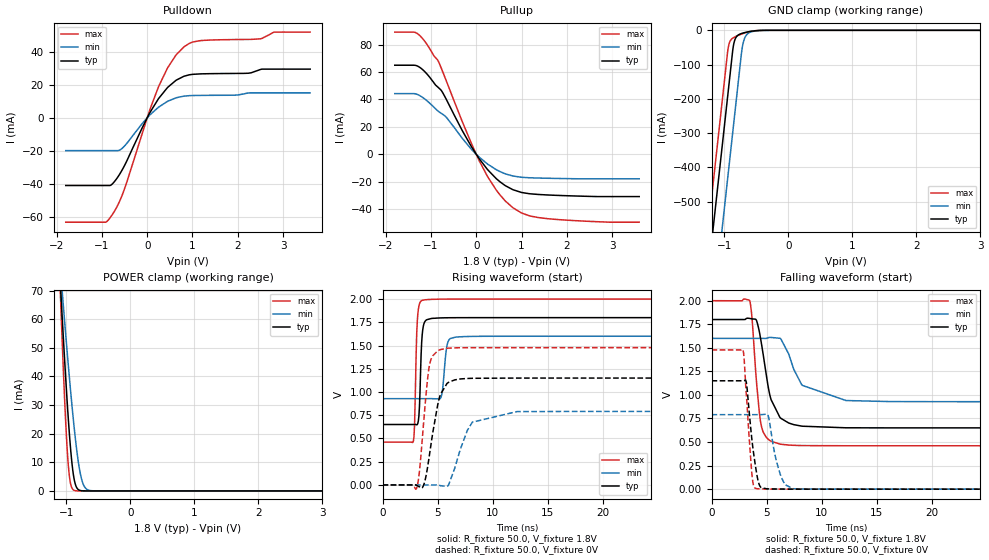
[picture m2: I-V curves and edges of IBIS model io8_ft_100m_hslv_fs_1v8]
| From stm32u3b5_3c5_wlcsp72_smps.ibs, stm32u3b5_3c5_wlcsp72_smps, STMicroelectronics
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[Model]   io8_ft_100m_hslv_fs_1v8
Model_type I/O
Polarity   Non-Inverting
Enable   Active-Low
| CAP_THRESHOLD on pad IOFT is "UDTCAPC" :
| Rising=30.0% of vddiom   Falling=70.0% of vddiom
| C_comp min and max val. don't necessarily correlate with the min and max pvt
| but are the smallest and greatest pad capacitance found.
| var   typ   min   max
C_comp   3.41787pF  3.41663pF  3.48192pF
|C_comp_pullup   1.92554pF  1.84326pF  2.10232pF
|C_comp_pulldown   1.49232pF  1.57337pF  1.37960pF
Vinl = 800.0mV
Vinh = 1.0V
Vmeas = 900.0mV   | Reference voltage for timing measurements
Cref  = 50.0pF   | Timing specification test load capacitance value
Rref  = 1.0MOhm   | Timing specification test load resistance value
Vref  = 990.0mV   | Timing specification test load voltage
[Model Spec]
| TIME_THRESHOLD on pin ZIV11 is "CMOS" :
| Rising=50.0% of vdd   Falling=50.0% of vdd
Vinl 694.50000mV 619.50000mV 778.50000mV
Vinh 1.08350V 957.50000mV 1.18750V
| variable   typ   min   max
[Temperature Range] 25.0 130.0 -40.0
| variable   typ   min   max
[Voltage Range] 1.8V 1.6V 2.0V
| variable   typ   min   max
[POWER Clamp Reference] 1.8V 1.6V 2.0V
| variable   typ   min   max
[GND Clamp Reference] 0V 0V 0V
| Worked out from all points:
|   slope of the pulldown table from 0 to 0.27 V, typ, clamps not added: 21.9 ohm
|   slope of the pullup table from 0 to 0.27 V, typ, clamps not added: 22.8 ohm
|   GND clamp passes 1 mA (typ) near -0.50 V on its own axis
|   POWER clamp passes 1 mA (typ) near -0.83 V on its own axis
|   rising waveform, R_fixture 50.0, V_fixture 1.8V: 20-80 % time 210ps typ, 321ps min, 196ps max; typ from 0.65 V to 1.8 V
|   falling waveform, R_fixture 50.0, V_fixture 1.8V: 20-80 % time 1.21ns typ, 2.33ns min, 635ps max; typ from 1.8 V to 0.65 V
|   rising waveform, R_fixture 50.0, V_fixture 0V: 20-80 % time 982ps typ, 1.45ns min, 660ps max; typ from 0 V to 1.15 V
|   falling waveform, R_fixture 50.0, V_fixture 0V: 20-80 % time 669ps typ, 867ps min, 510ps max; typ from 1.15 V to 0 V
[POWER Clamp]
-1.8V     399.1mA    292.1mA    557.7mA
-1.09V    71.2mA     76.8mA     67.14mA
-1.08V    67.05mA    73.98mA    61.2mA
-1.06V    58.89mA    68.38mA    49.67mA
-1.02V    43.22mA    57.4mA     28.67mA
-980mV    28.81mA    46.77mA    12.28mA
-940mV    16.45mA    36.61mA    3.257mA
-880mV    4.35mA     22.67mA    225.4uA
-820mV    610.4uA    11.29mA    13uA
-770mV    97.5uA     4.87mA     1.193uA
-640mV    753.9nA    196uA      2.492nA
3.6V      0A         0A         0A
[GND Clamp]
-1.8V     -1.64A     -1.88A     -1.509A
-1.24V    -688.2mA   -927.9mA   -557mA
-1.05V    -365.2mA   -604.9mA   -234mA
-950mV    -195.2mA   -434.9mA   -64mA
-930mV    -161.2mA   -400.9mA   -41.59mA
-870mV    -59.19mA   -298.9mA   -22.94mA
-850mV    -36.73mA   -264.9mA   -20.65mA
-770mV    -12.21mA   -128.9mA   -13.73mA
-730mV    -9.139mA   -62.1mA    -10.81mA
-690mV    -6.97mA    -26.33mA   -8.198mA
-530mV    -1.564mA   -2.413mA   -1.407mA
3.6V      1.228nA    159.5nA    526.9pA
| variable   typ   min   max
[Pullup Reference] 1.8V 1.6V 2.0V
| variable   typ   min   max
[Pulldown Reference] 0V 0V 0V
[Pullup]
-1.8V     64.92mA    44.22mA    89.08mA
-1.3V     64.34mA    43.62mA    87.96mA
-1.13V    59.98mA    40.13mA    82.03mA
-850mV    49.04mA    31.68mA    68.55mA
-670mV    40.59mA    27.29mA    54.24mA
-310mV    17.35mA    11.71mA    23.94mA
70mV      -3.42mA    -2.198mA   -4.946mA
440mV     -17.67mA   -11.15mA   -25.97mA
810mV     -25.79mA   -15.81mA   -38.95mA
1.18V     -28.75mA   -17.1mA    -44.89mA
1.56V     -29.61mA   -17.45mA   -46.86mA
3.6V      -30.8mA    -17.88mA   -49.48mA
[Pulldown]
-1.8V     -41.16mA   -19.96mA   -63.43mA
-920mV    -41.16mA   -19.96mA   -63.43mA
-780mV    -40.43mA   -19.96mA   -59.18mA
-510mV    -29.46mA   -17.38mA   -43.8mA
0V        0A         -230fA     0A
250mV     11.64mA    6.428mA    18.87mA
460mV     18.67mA    10.12mA    30.76mA
810mV     25.21mA    13.14mA    43.03mA
1.18V     26.67mA    13.59mA    46.9mA
2.5V      29.31mA    15.12mA    47.95mA
2.81V     29.55mA    15.12mA    52.03mA
3.6V      29.55mA    15.12mA    52.05mA
[Ramp]
dV/dt_r 690.0298mV/981.32916ps 474.38109mV/1.40579ns 886.36843mV/658.85282ps
dV/dt_f 689.75447mV/1.12579ns 403.00076mV/1.68065ns 923.68055mV/633.67172ps
R_load = 50.0
| Removed startup time: 0s 0s 0s  .
| Removed end time: 36.25ns.
[Rising Waveform]
R_fixture   = 50.0
V_fixture   = 1.8V
V_fixture_min = 1.6V
V_fixture_max = 2.0V
0s        650.4mV    928.3mV    460.5mV
2.8ns     650.7mV    928.3mV    473mV
2.9ns     650.8mV    928.3mV    632mV
3.15ns    649.8mV    928.3mV    1.755V
3.35ns    842.4mV    928.3mV    1.948V
3.6ns     1.617V     928.3mV    1.986V
5.25ns    1.797V     930.7mV    1.999V
5.9ns     1.799V     1.525V     2V
6.65ns    1.8V       1.591V     2V
36.25ns   1.8V       1.6V       2V
| Removed startup time: 0s 0s 0s  .
| Removed end time: 199.25ns.
[Falling Waveform]
R_fixture   = 50.0
V_fixture   = 1.8V
V_fixture_min = 1.6V
V_fixture_max = 2.0V
0s        1.8V       1.6V       2V
3.45ns    1.812V     1.6V       2.003V
3.65ns    1.808V     1.6V       1.842V
4.05ns    1.797V     1.6V       1.178V
4.55ns    1.527V     1.6V       655.8mV
5.4ns     950.1mV    1.61V      508.8mV
7ns       702mV      1.435V     468mV
8.25ns    668mV      1.101V     462.5mV
16.25ns   650.5mV    929.4mV    460.5mV
199.3ns   650.4mV    928.3mV    460.5mV
| Removed startup time: 0s 0s 0s  .
| Removed end time: 199.2ns.
[Rising Waveform]
R_fixture   = 50.0
V_fixture   = 0V
V_fixture_min = 0V
V_fixture_max = 0V
0s        4.636nV    97.72nV    3.408nV
3.05ns    -1.213mV   -226.6nV   -44.13mV
3.3ns     -17.75mV   -1.125uV   96.7mV
3.7ns     -9.956mV   -9.028uV   631mV
4.3ns     357.9mV    -18.37uV   1.312V
5.15ns    933.4mV    -2.891mV   1.452V
6ns       1.105V     2.808mV    1.472V
8.15ns    1.148V     675.6mV    1.477V
12.2ns    1.15V      789.4mV    1.477V
199.2ns   1.15V      790.6mV    1.477V
| Removed startup time: 0s 0s 0s  .
| Removed end time: 36.25ns.
[Falling Waveform]
R_fixture   = 50.0
V_fixture   = 0V
V_fixture_min = 0V
V_fixture_max = 0V
0s        1.15V      790.6mV    1.477V
2.85ns    1.15V      790.6mV    1.481V
3.15ns    1.136V     790.6mV    1.007V
3.65ns    536.3mV    790.6mV    171.8mV
4.05ns    195.9mV    790.7mV    6.559mV
4.4ns     30.04mV    790.7mV    3.072mV
5.1ns     3.457mV    790.2mV    1.414mV
6.3ns     1.163mV    133.8mV    471.6uV
7.4ns     526uV      4.771mV    194.6uV
36.25ns   48.37nV    588.8nV    5.956nV
